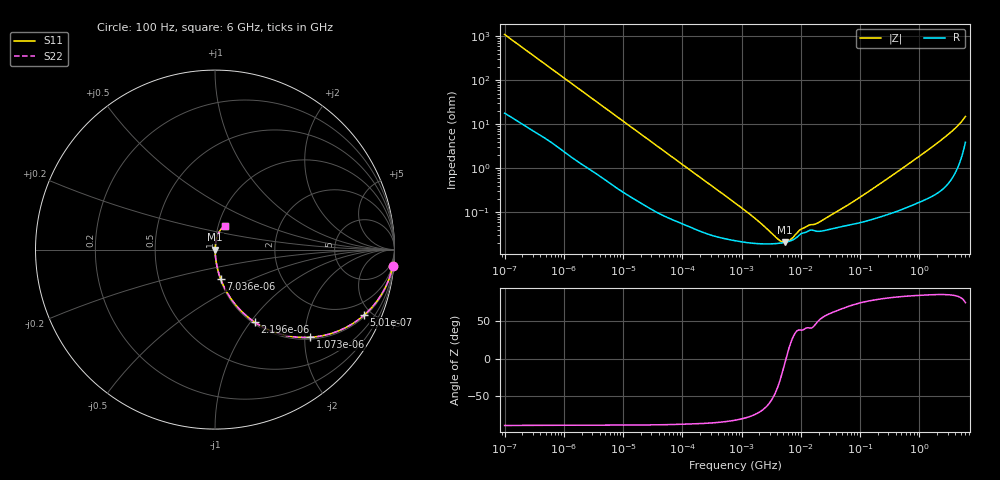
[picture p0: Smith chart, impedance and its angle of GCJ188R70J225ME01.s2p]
!Murata Part Number: GCJ188R70J225ME01
!These Parameters are Measured in Series Mode Connection
!Data Generated on Mar 13, 2026
!  o--ll--o
!Port1  Port2
!  o------o
!Operation Temp=25[degC], DC Bias Voltage=0[V]
!Freq. Start=100[Hz] Stop=6[GHz] 401[Steps]
# Hz S RI R 50
!Freq.(Hz) S11(Real) S11(Imag) S21(Real) S21(Imag) S12(Real) S12(Imag) S22(Real) S22(Imag)
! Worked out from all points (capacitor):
!   401 points, 100 Hz to 6 GHz, reference 50 ohm
!   read as one part in series: C = 1.43 uF near 109 Hz
!   lowest |Z| = 20.7 mohm at 5.312 MHz (marker M1)
!   series resonance near 5.612 MHz, so ESL is about 560 pH
!   S11 on the Smith chart (normalised r, x): 100 Hz: 1, -22; 501 Hz: 1.09, -4.52; 1.073 kHz: 1.04, -2.13; 2.196 kHz: 1.02, -1.05; 7.036 kHz: 1.01, -0.33; 6 GHz: 1.08, +0.29
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100  0.9905 -0.089  0.00945 0.089  0.00945 0.089  0.9905 -0.089
268  0.9425 -0.2236  0.0575 0.2236  0.0575 0.2236  0.9425 -0.2236
501  0.8313 -0.3643  0.1687 0.3643  0.1687 0.3643  0.8313 -0.3643
1073  0.532 -0.4886  0.468 0.4886  0.468 0.4886  0.532 -0.4886
2008  0.253 -0.4241  0.747 0.4241  0.747 0.4241  0.253 -0.4241
2196  0.2218 -0.4048  0.7782 0.4048  0.7782 0.4048  0.2218 -0.4048
3759  0.0929 -0.279  0.9071 0.279  0.9071 0.279  0.0929 -0.279
7036  0.0307 -0.1613  0.9693 0.1613  0.9693 0.1613  0.0307 -0.1613
15062  0.00817 -0.078  0.9918 0.078  0.9918 0.078  0.00817 -0.078
40335  0.00183 -0.0298  0.9982 0.0298  0.9982 0.0298  0.00183 -0.0298
774597  0.000228 -0.00162  0.9998 0.00162  0.9998 0.00162  0.000228 -0.00162
1896632  0.000194 -0.000608  0.9998 0.000608  0.9998 0.000608  0.000194 -0.000608
4060267  0.000196 -0.000154  0.9998 0.000154  0.9998 0.000154  0.000196 -0.000154
5311619  0.000206 -2.57e-05  0.9998 2.57e-05  0.9998 2.57e-05  0.000206 -2.57e-05
6644369  0.000223 8.03e-05  0.9998 -8.03e-05  0.9998 -8.03e-05  0.000223 8.03e-05
9941735  0.00032 0.000254  0.9997 -0.000254  0.9997 -0.000254  0.00032 0.000254
1.555665e7  0.000392 0.000348  0.9996 -0.000348  0.9996 -0.000348  0.000392 0.000348
1.946e7  0.000368 0.00044  0.9996 -0.00044  0.9996 -0.00044  0.000368 0.00044
5.699437e7  0.000494 0.00127  0.9995 -0.00127  0.9995 -0.00127  0.000494 0.00127
3.124326e8  0.000951 0.00615  0.999 -0.00615  0.999 -0.00615  0.000951 0.00615
2.34314e9  0.00503 0.0436  0.995 -0.0436  0.995 -0.0436  0.00503 0.0436
6e9  0.0563 0.1329  0.9437 -0.1329  0.9437 -0.1329  0.0563 0.1329
